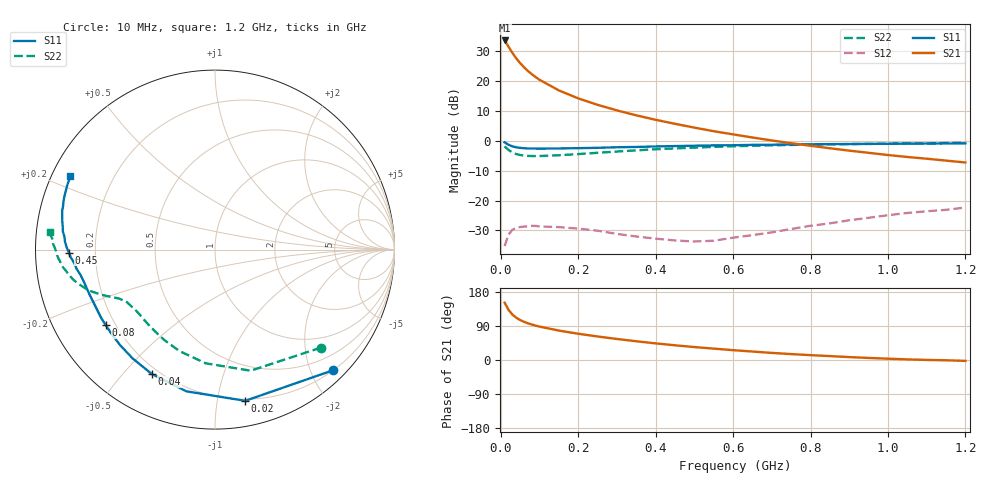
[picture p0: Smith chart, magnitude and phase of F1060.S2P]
! Date: Tue Aug 08 10:36:13 1995
# MHZ  S  MA  R  50.0000
!  POLYFET RF DEVICES
!  F1060
!  S PARAMETERS
!  VDS=28V, IDQ=200mA
!FREQ  S11MAG S11ANG S21MAG S21ANG S12MAG S12ANG S22MAG S22ANG
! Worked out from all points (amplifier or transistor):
!   32 points, 10 MHz to 1.2 GHz, reference 50 ohm
!   highest |S21| = 33.6 dB at 10 MHz (marker M1)
!   |S21| within 3 dB of that: start of sweep to 24.5 MHz
!   unconditionally stable (mu >= 1): 344 MHz to 773.8 MHz
!   at 60 MHz: K = 0.15, MSG = 26.7 dB, |S12| = -28.7 dB
!   at 450 MHz: K = 1.35, MAG = 16.0 dB, |S12| = -33.4 dB
!   at 1.2 GHz: K = 0.51, MSG = 7.5 dB, |S12| = -22.3 dB
!   S11 on the Smith chart (normalised r, x): 10 MHz: 0.21, -2.36; 20 MHz: 0.19, -1.20; 40 MHz: 0.17, -0.60; 80 MHz: 0.16, -0.30; 450 MHz: 0.10, -0.01; 1.2 GHz: 0.05, +0.24
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10  0.9396 -45.7  47.72 151.4  0.01721 63.4  0.8039 -42.8
20  0.8591 -78.7  37.6 132.4  0.02681 45.5  0.7034 -73.6
30  0.8055 -101.4  29.64 120.0  0.03239 32.8  0.6357 -94.6
40  0.7775 -116.9  23.92 111.6  0.03461 26.0  0.5991 -109.3
50  0.7604 -127.1  19.99 105.6  0.03595 20.4  0.5776 -119.3
60  0.7502 -135.0  17.03 100.8  0.03664 15.8  0.5644 -126.7
70  0.7436 -140.7  14.76 96.9  0.0368 13.3  0.5582 -132.2
80  0.7398 -145.3  13.05 93.6  0.03766 10.6  0.5551 -136.2
90  0.7399 -148.9  11.64 90.8  0.03757 9.1  0.5542 -139.3
100  0.7377 -151.9  10.5 88.2  0.03692 7.6  0.5553 -141.8
150  0.7436 -161.1  6.97 77.7  0.03587 2.1  0.5717 -149.2
200  0.7518 -166.0  5.126 69.3  0.03386 -1.7  0.5985 -152.8
250  0.7626 -169.4  3.995 62.1  0.03124 -2.2  0.6289 -155.1
300  0.7783 -172.0  3.223 55.5  0.0276 -1.1  0.6603 -157.0
350  0.7874 -174.5  2.664 49.5  0.025 1.6  0.6907 -159.0
400  0.8032 -176.7  2.244 43.8  0.023 8.2  0.7211 -160.9
450  0.8147 -178.9  1.921 38.8  0.02143 16.5  0.745 -162.6
550  0.8372 176.9  1.444 30.0  0.02121 37.7  0.7903 -166.5
650  0.8537 173.2  1.133 22.3  0.02633 50.7  0.8236 -169.9
850  0.8785 165.7  0.7485 10.3  0.04148 65.8  0.872 -176.5
1050  0.8936 158.4  0.5352 1.7  0.0619 66.6  0.9024 178.0
1200  0.9042 153.0  0.4331 -2.4  0.07632 64.7  0.9223 174.0
